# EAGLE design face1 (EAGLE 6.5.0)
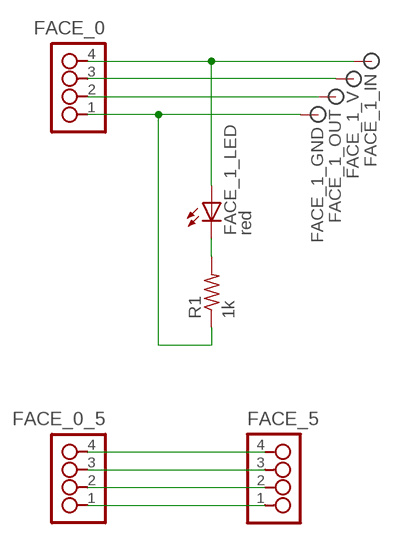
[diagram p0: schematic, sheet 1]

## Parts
FACE_0  4_PIN_HEADER  [SMT_PINS_4]
FACE_0_5  4_PIN_HEADER  [SMT_PINS_4]
FACE_1_GND  SIGNAL  [PAD.2]
FACE_1_IN  SIGNAL  [PAD.2]
FACE_1_LED  red  LED1206  [1206]
FACE_1_OUT  SIGNAL  [PAD.2]
FACE_1_V  SIGNAL  [PAD.2]
FACE_5  4_PIN_HEADER  [SMT_PINS_4]
R1  1k  RESISTOR1206  [1206]

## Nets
GND: FACE_0.1 FACE_1_GND.P$1 R1.1
IN: FACE_0.4 FACE_1_IN.P$1 FACE_1_LED.1(A)
N$5: FACE_1_LED.2(C) R1.2
N$6: FACE_0_5.4 FACE_5.4
N$7: FACE_0_5.3 FACE_5.3
N$8: FACE_0_5.2 FACE_5.2
N$9: FACE_0_5.1 FACE_5.1
OUT: FACE_0.2 FACE_1_OUT.P$1
V: FACE_0.3 FACE_1_V.P$1

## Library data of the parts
FACE_0 FACE_0_5 FACE_5 = ot:4_PIN_HEADER
FACE_1_GND FACE_1_IN FACE_1_OUT FACE_1_V = ot:SIGNAL: Signal
FACE_1_LED = 01_FAB_Hello:LED
R1 = 01_FAB_Hello:RESISTOR

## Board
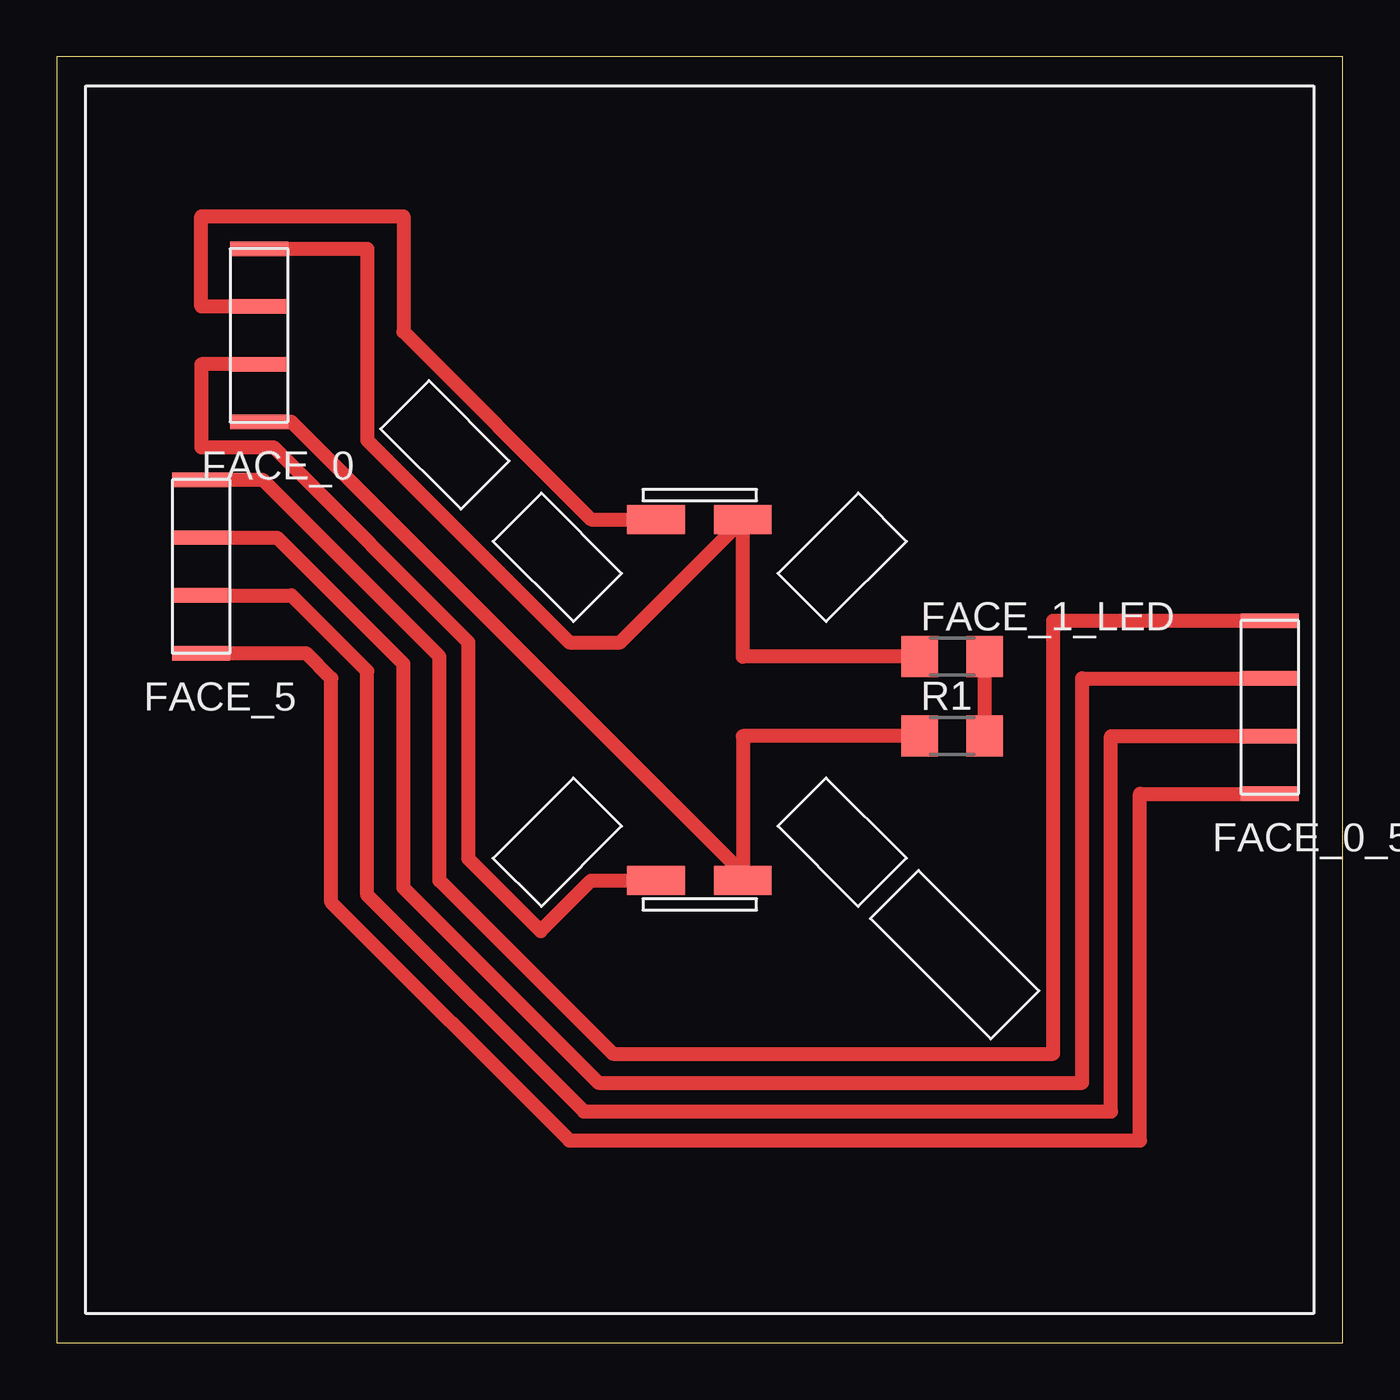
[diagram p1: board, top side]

Size 56.54 x 56.54 mm. Coordinates in mm from the lower left corner, seen from the top.
Outline: 0,0 56.54,0 56.54,56.54 0,56.54 0,0
Copper layers (1*16): Top 0.035mm / dielectric 1.5mm / Bottom 0.035mm
Design rules "default": minimum track width 10mil, minimum drill 24mil, track to track 8mil, track to pad 8mil, pad to pad 8mil, via to via 8mil, smd to smd 8mil, copper to edge 40mil, drill to drill 8mil, minimum pad ring 10mil, minimum via ring 8mil, stop-mask expansion 4mil, vias tented up to drill 0mil, thermal gap 10mil

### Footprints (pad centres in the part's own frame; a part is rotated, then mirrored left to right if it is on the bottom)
SMT_PINS_4 = smd 2.54 x 0.635: 1 0,0; 2 0,2.54; 3 0,5.08; 4 0,7.62
PAD.2 = smd 2.54 x 1.27: P$1 0,0
1206 = smd 1.6 x 1.803: 1 -1.422,0; 2 1.422,0

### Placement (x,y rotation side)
FACE_0  8.89,40.48 0 top
FACE_0_5  53.34,24.13 0 top
FACE_1_GND  30.16,20.32 0 top
FACE_1_IN  30.16,36.2 0 top
FACE_1_LED  39.37,30.16 0 top
FACE_1_OUT  26.35,20.32 0 top
FACE_1_V  26.35,36.2 0 top
FACE_5  6.35,30.32 0 top
R1  39.37,26.67 0 top
U$1  [CUBE_NEG]  1.27,55.27 270 top

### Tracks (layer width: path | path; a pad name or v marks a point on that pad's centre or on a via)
GND
  Top 0.61: R1.1 30.16,26.67 FACE_1_GND.P$1 30.16,20.64 10.32,40.48 FACE_0.1
IN
  Top 0.61: FACE_0.4 13.65,48.1 13.65,39.69 22.54,30.8 24.77,30.8 FACE_1_IN.P$1 30.16,30.16 FACE_1_LED.1
N$5
  Top 0.61: FACE_1_LED.2 R1.2
N$6
  Top 0.61: FACE_5.4 9.05,37.94 16.83,30.16 16.83,20.32 24.45,12.7 43.81,12.7 43.81,31.75 FACE_0_5.4
N$7
  Top 0.61: FACE_5.3 9.68,35.4 15.24,29.84 15.24,20 23.81,11.43 45.09,11.43 45.09,29.21 FACE_0_5.3
N$8
  Top 0.61: FACE_5.2 10.32,32.86 13.65,29.53 13.65,19.68 23.18,10.16 46.35,10.16 46.35,26.67 FACE_0_5.2
N$9
  Top 0.61: FACE_5.1 10.95,30.32 12.06,29.21 12.06,19.37 22.54,8.89 47.62,8.89 47.62,24.13 FACE_0_5.1
OUT
  Top 0.61: FACE_0.2 6.35,43.02 6.35,39.37 9.53,39.37 18.1,30.8 18.1,21.27 21.27,18.1 23.5,20.32 FACE_1_OUT.P$1
V
  Top 0.61: FACE_0.3 6.35,45.56 6.35,49.53 15.24,49.53 15.24,44.45 23.5,36.2 FACE_1_V.P$1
